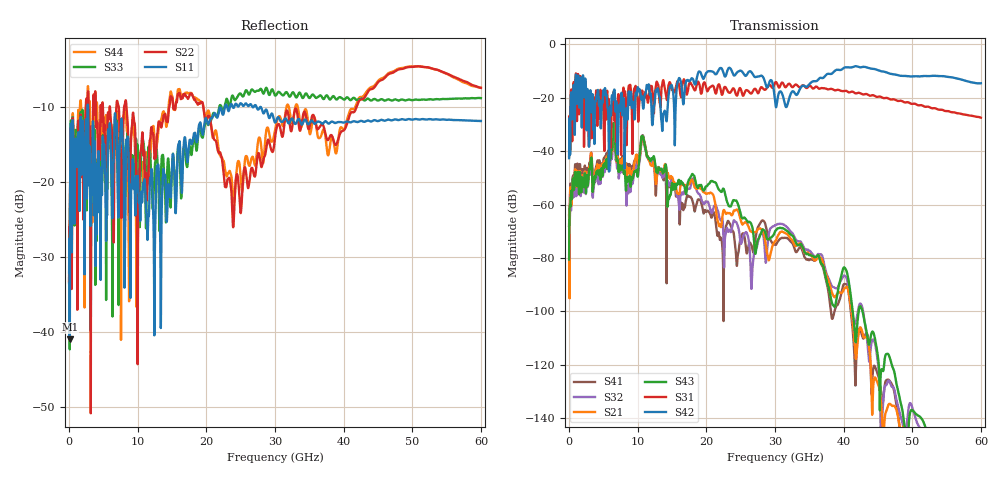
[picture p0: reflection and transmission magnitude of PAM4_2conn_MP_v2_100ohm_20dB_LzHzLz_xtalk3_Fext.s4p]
! Info: Touchstone file created by Circ.  Input file=FAB50GbE_2conn_Midplane_Examax_Topo2_v2_100ohm_20dB_LzHzLz.circ
# Hz S RI R 50
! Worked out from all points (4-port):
!   6000 points, 10 MHz to 60 GHz, reference 50 ohm
!   strongest paths, dB at 10 MHz, 15.01 GHz, 30.01 GHz, 45.01 GHz, 60 GHz:
!     S42: -42.6, -15.7, -21.2, -9.7, -14.6
!     S31: -41.9, -17.1, -14.4, -19.7, -27.5
!     S43: -80.6, -51.9, -70.1, -117.1, -159.3
!     S21: -64.1, -49.8, -73.7, -127.2, -165.2
!     S32: -68.1, -50.3, -67.7, -119.4, -164.9
!     S41: -67.5, -52.1, -75.0, -123.8, -176.5
!   lowest |S11| = -41.0 dB at 100 MHz (marker M1), VSWR 1.02, Z = 50.2 - j0.87 ohm
!   |S11| at or under -10 dB: start of sweep to 2.7 GHz; 2.752 GHz to 22.7 GHz (19.95 GHz wide, 157 % of centre); 27.97 GHz to end of sweep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
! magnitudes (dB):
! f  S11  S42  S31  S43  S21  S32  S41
! 10 MHz  -32.0  -42.6  -41.9  -80.6  -64.1  -68.1  -67.5
! 100 MHz  -41.0  -28.2  -27.4  -60.4  -69.5  -66.0  -64.4
! 1.18 GHz  -17.9  -20.2  -20.6  -48.9  -47.7  -50.1  -45.4
! 6.47 GHz  -17.4  -18.2  -19.0  -29.7  -31.6  -33.7  -29.8
! 24.48 GHz  -9.7  -10.5  -19.2  -59.1  -61.9  -67.3  -82.4
! 27.22 GHz  -9.8  -12.2  -16.9  -77.4  -70.3  -76.5  -71.7
! 60 GHz  -11.8  -14.6  -27.5  -159.3  -165.2  -164.9  -176.5
